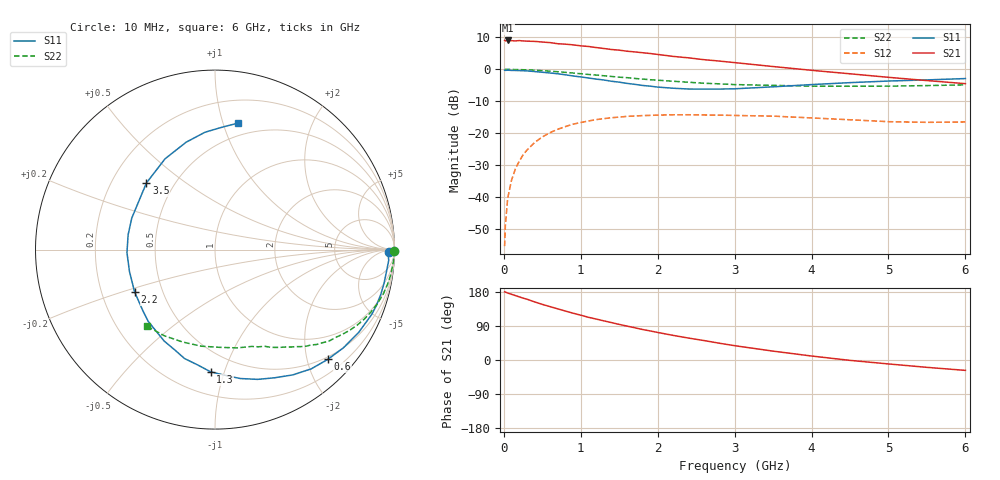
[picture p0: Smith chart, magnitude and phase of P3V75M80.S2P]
! SIEMENS Small Signal Semiconductors
! BFP181
! Si NPN RF Bipolar Junction Transistor in SOT143
! VCE = 0.75 V  IC = 0.8 mA
! Common Emitter S-Parameters:  March  1996
# GHz  S  MA  R  50
!  f  S11  S21  S12  S22
! GHz  MAG  ANG  MAG  ANG  MAG  ANG  MAG  ANG
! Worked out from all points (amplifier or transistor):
!   36 points, 10 MHz to 6 GHz, reference 50 ohm
!   highest |S21| = 9.1 dB at 50 MHz (marker M1)
!   |S21| within 3 dB of that: start of sweep to 1.482 GHz
!   unconditionally stable (mu >= 1): 2.999 GHz to end of sweep
!   at 250 MHz: K = 0.09, MSG = 17.9 dB, |S12| = -26.8 dB
!   at 1.4 GHz: K = 0.51, MSG = 10.7 dB, |S12| = -15.2 dB
!   at 6 GHz: K = 1.47, MAG = 1.9 dB, |S12| = -16.5 dB
!   S11 on the Smith chart (normalised r, x): 10 MHz: 50, -24; 600 MHz: 0.45, -2.39; 1.3 GHz: 0.35, -0.90; 2.2 GHz: 0.35, -0.22; 3.5 GHz: 0.35, +0.36; 6 GHz: 0.39, +1.13
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0.01  0.9682 -0.9  2.834 179.7  0.0017 89.3  0.9983 -0.3
0.02  0.964 -1.4  2.8 179.4  0.0036 85.6  0.9976 -0.8
0.05  0.9698 -3.5  2.835 176.7  0.0096 88.0  0.9967 -1.9
0.1  0.963 -7.5  2.812 173.4  0.0184 84.1  0.9964 -3.8
0.15  0.9603 -11.4  2.789 170.0  0.0276 82.5  0.9922 -5.7
0.2  0.9569 -15.1  2.821 166.6  0.0363 79.6  0.9902 -7.5
0.25  0.9519 -18.9  2.787 163.2  0.0457 77.5  0.9858 -9.4
0.4  0.9242 -29.9  2.742 153.3  0.0714 69.8  0.9694 -14.9
0.6  0.877 -44.2  2.623 140.9  0.102 59.9  0.9365 -21.8
0.9  0.7879 -65.0  2.42 123.5  0.1385 47.0  0.8763 -30.7
1.1  0.7319 -78.9  2.282 112.7  0.1554 39.5  0.8321 -36.0
1.3  0.6813 -92.1  2.122 103.3  0.169 32.3  0.7935 -40.8
1.5  0.6303 -105.6  1.999 93.9  0.1787 26.5  0.7539 -44.8
1.8  0.5602 -125.9  1.823 80.6  0.1886 19.1  0.7046 -50.1
2.2  0.5062 -152.2  1.595 65.0  0.1942 9.9  0.6513 -56.8
2.4  0.492 -165.6  1.515 57.9  0.1945 5.9  0.6283 -60.1
2.8  0.491 170.3  1.349 44.3  0.1919 -0.2  0.5933 -65.9
3.5  0.5328 135.8  1.107 23.4  0.1851 -8.8  0.5614 -77.3
4  0.5774 118.8  0.966 10.5  0.1734 -13.0  0.5452 -87.2
4.5  0.6194 105.1  0.852 -1.0  0.1623 -16.1  0.5436 -98.1
5.5  0.6835 86.6  0.667 -19.4  0.1479 -14.0  0.5569 -120.4
6  0.7173 79.5  0.597 -27.4  0.1499 -11.9  0.5711 -131.8
